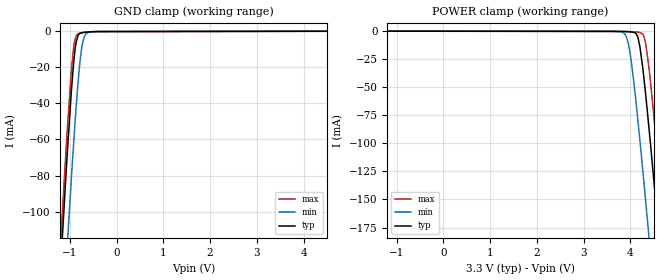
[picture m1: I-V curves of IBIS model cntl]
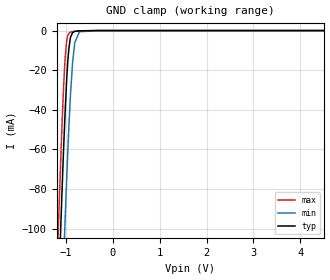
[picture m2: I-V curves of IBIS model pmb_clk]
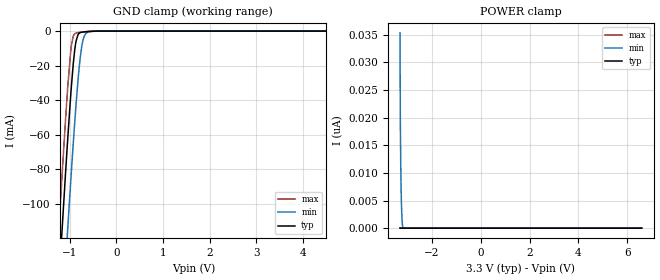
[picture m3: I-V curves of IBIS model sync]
|Texas Instruments Incorporated
| TPS40400 3.0-V TO 20-V PMBus SYNCHRONOUS BUCK CONTROLLER
| Marketing part#   Digital Voltage Range   Package-type   #pins
| TPS40400RHLR   3.0V-3.4V   VQFN   24
| TPS40400RHLT   3.0V-3.4V   VQFN   24
[IBIS Ver]   4.1
[File name]   tps40400.ibs
[File Rev]   2.0
[Date]   4/17/2015
[Source]
| Texas Instruments Incorporated.
| Analog-eLab Design Center, HPA
| 12500 TI Blvd
| Dallas, TX -75243
[Notes]   Revision History:
| Rev 2.0: 4/17/2015
| - New models added for CNTL, PGOOD and SYNC.
| Rev 1.1: 7/1/2013
| - Modeled with respect to different V_fixture voltages
| Rev 1.0: 6/21/2013
| - Initial version of the model
| - Model generated from simulations in TISPICE
| - Model matched to SPICE simulation
| - C_comp although listed in numerical order of value are
|   obtained from varying PVT conditions. For PVT conditions for
|   each specific value refer the buffer description under
|   respective [Model]. IBIS model user is responsible for using
|   appropriate C_comp to simulate for Signal Integrity.
|*  EXCEPTION:   *
|*  - For model sync, there will be a leakage current in the Ground Clamp   *
|*   I-V Table because of the pulldown transistors MN0 and MN1 in ESD   *
|*   connected to pad.   *
|*  - For model pgood, there will be a leakage current in the Power Clamp   *
|*   I-V Table because of the MP1 and MN1 transistors in the BU140 block   *
|*   connected to pad.End points do not match fixture voltages due to the   *
|*   pull up resistance (100kohms)  connected to the pad.   *
|*  - For model smbalrt, there will be a leakage current in the Power Clamp  *
|*   I-V Table because of the transistor MN1 in PGOOD_FET block connected   *
|*   to pad.   *
|*  - For model data, there will be a leakage current in the Power Clamp   *
|*   I-V Table because of the transistor (MN0, MN1) and diode (XDD0) in   *
|*   ESD block  connected to pad.   *
[Disclaimer]
| This model is designed as an aid for customers of Texas Instruments.
| TI and its licensors and suppliers make no warranties, either expressed
| or implied, with respect to this  model, including the warranties of
| merchantability or fitness for a particular purpose. The model is
| provided solely on an "as is" basis. The entire risk as to its quality
| and performance is with the customer.
[Copyright]
(C) Copyright 2015 Texas Instruments Incorporated.All rights reserved.
|   TPS540400
[Component]   TPS540400
[Manufacturer]   TI
[Package]   |24 VQFN
|   typ   min   max
R_pkg  0.042266   0.000540  0.065360
L_pkg  0.707532nH 0.114770nH 1.090470nH
C_pkg  0.120390pF 0.069160pF 0.145430pF
[Pin]  signal_name   model_name   R_pin   L_pin   C_pin
1   CLK   pmb_clk   NA   NA   NA
2   CNTL   cntl   NA   NA   NA
3   PGOOD   pgood   NA   NA   NA
4   SYNC   sync   NA   NA   NA
5   TRACK   NC   NA   NA   NA
6   COMP   NC   NA   NA   NA
7   FB   NC   NA   NA   NA
8   DIFFO   NC   NA   NA   NA
9   VSNS+   NC   NA   NA   NA
10   VSNS-   NC   NA   NA   NA
11   ISNS-   NC   NA   NA   NA
12   ISNS+   NC   NA   NA   NA
13   BP3   NC   NA   NA   NA
14   BP6   NC   NA   NA   NA
15   GND   GND   NA   NA   NA
16   LDRV   NC   NA   NA   NA
17   SW   NC   NA   NA   NA
18   BOOT   NC   NA   NA   NA
19   HDRV   NC   NA   NA   NA
20   VDD   POWER   NA   NA   NA
21   ADDR0   nc   NA   NA   NA
22   ADDR1   nc   NA   NA   NA
23   SMBALRT   smbalrt   NA   NA   NA
24   DATA   data   NA   NA   NA
|   Model Selectors
[Model Selector] data
data_pr_5   3.3V digital I/O_open_drain with V_fixture = 5V
data_pr_3p3 3.3V digital I/O_open_drain with V_fixture = 3.3V
data_pr_1p8 3.3V digital I/O_open_drain with V_fixture = 1.8V
[Model Selector] smbalrt
smbalrt_pr_5   3.3V digital open_sink with V_fixture = 5V
smbalrt_pr_3p3 3.3V digital open_sink with V_fixture = 3.3V
smbalrt_pr_1p8 3.3V digital open_sink with V_fixture = 1.8V
[Model Selector] pgood
pgood_pr_5   3.3V digital open_sink with V_fixture = 5V
pgood_pr_3p3 3.3V digital open_sink with V_fixture = 3.3V
pgood_pr_1p8 3.3V digital open_sink with V_fixture = 1.8V
| Models and submodels in the file (12): cntl (Input), pmb_clk (Input), sync (Input), smbalrt_pr_1p8 (Open_sink), smbalrt_pr_3p3 (Open_sink), smbalrt_pr_5 (Open_sink), data_pr_1p8 (I/O_open_drain), data_pr_3p3 (I/O_open_drain), data_pr_5 (I/O_open_drain), pgood_pr_5 (Open_drain), pgood_pr_3p3 (Open_drain), pgood_pr_1p8 (Open_drain)
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|   cntl Model
[Model]   cntl
Model_type   Input
Vinl = 0.8
Vinh = 2.1
|   typ   min   max
C_comp   0.176pF   0.150pF   0.210pF
[Voltage Range]   3.3   3.2   3.4
[Temperature Range]   25   125   -40
[Power Clamp Reference]   3.3   3.2   3.4
[GND Clamp Reference]   -0   -0   -0
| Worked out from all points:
|   GND clamp passes 1 mA (typ) near -0.73 V on its own axis
[GND Clamp]
|   Voltage   I(typ)   I(min)   I(max)
-3.3V     -1.154A    -1.202A    -1.142A
-1.231V   -146.1mA   -198.6mA   -132.5mA
-1.092V   -84.06mA   -135.8mA   -70.75mA
-1.043V   -63.1mA    -114.1mA   -50.17mA
-973.5mV  -35.96mA   -84.64mA   -24.42mA
-924mV    -19.54mA   -64.6mA    -10.6mA
-864.6mV  -6.393mA   -42.31mA   -2.848mA
-815.1mV  -2.251mA   -26.11mA   -1.478mA
-755.7mV  -1.16mA    -11.44mA   -1.108mA
-706.2mV  -923.4uA   -4.598mA   -948.2uA
-547.8mV  -553.6uA   -646.5uA   -584.9uA
6.59V     -180.4uA   -165uA     -204.1uA
[POWER Clamp]
|   Voltage   I(typ)   I(min)   I(max)
-3.3V     -180uA     -168.1uA   -199.9uA
3.818V    -509.1uA   -1.084mA   -476.1uA
3.917V    -688.3uA   -5.682mA   -541.7uA
3.986V    -861.9uA   -18.23mA   -654.3uA
4.125V    -2.705mA   -64.99mA   -1.004mA
4.204V    -14.18mA   -97.53mA   -1.371mA
4.293V    -43.35mA   -136.3mA   -5.351mA
4.333V    -59.03mA   -154mA     -12.65mA
4.402V    -88.35mA   -185.4mA   -34.47mA
4.6V      -178.2mA   -277.5mA   -118.5mA
4.788V    -266.9mA   -366.7mA   -206mA
6.59V     -1.149A    -1.247A    -1.087A
|   pmb_clk Model
[Model]   pmb_clk
Model_type   Input
Vinl = 0.8
Vinh = 2.1
|   typ   min   max
|   (nom PVT)   (fast PVT)   (slow PVT)
C_comp   5.652e-14   5.542e-14   5.833e-14
| Where nom  PVT is Nominal Process, 3.3V, 25C
|   Fast PVT is Strong Process,  3.4V, -40C
|   Slow PVT is Weak Process,   3.2V, 125C
[Voltage Range]   3.3   3.2   3.4
|Junction Temperature
[Temperature Range]   25   125   -40
[Power Clamp Reference]   3.3   3.2   3.4
[GND Clamp Reference]   0   0   0
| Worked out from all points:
|   GND clamp passes 1 mA (typ) near -0.85 V on its own axis
[GND Clamp]
|   Voltage   I(typ)   I(min)   I(max)
-3.3V     -1.871A    -1.918A    -1.848A
-1.175V   -145.3mA   -205mA     -109.9mA
-1.158V   -133.2mA   -192.9mA   -97.97mA
-1.143V   -122.5mA   -182mA     -87.34mA
-1.09V    -85.9mA    -144.4mA   -51.94mA
-1.025V   -45.95mA   -101.1mA   -17.51mA
-960.8mV  -16mA      -61.8mA    -2.658mA
-904.2mV  -3.714mA   -33.19mA   -823.8uA
-858.4mV  -1.052mA   -16.34mA   -532uA
-813.6mV  -421.3uA   -6.609mA   -368.5uA
-711.2mV  -114.9uA   -593.5uA   -127.1uA
6.6V      0A         0A         0A
[POWER Clamp]
|   Voltage   I(typ)   I(min)   I(max)
-3.3V     0A         0A         0A
0V        0A         0A         0A
6.6V      0A         0A         0A
|   sync Model
[Model]   sync
Model_type   Input
Vinl = 0.8
Vinh = 2.1
|   typ   min   max
C_comp   0.254pF   0.192pF   0.296pF
[Voltage Range]   3.3   3.2   3.4
[Temperature Range]   25   125   -40
[Power Clamp Reference]   3.3   3.2   3.4
[GND Clamp Reference]   -0   -0   -0
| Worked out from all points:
|   GND clamp passes 1 mA (typ) near -0.78 V on its own axis
[GND Clamp]
|   Voltage   I(typ)   I(min)   I(max)
-3.3V     -1.153A    -1.202A    -1.125A
-1.27V    -163.3mA   -216.8mA   -131.5mA
-1.231V   -145.1mA   -198.6mA   -113.2mA
-1.181V   -122.5mA   -175.9mA   -90.69mA
-1.043V   -62.05mA   -114.1mA   -32.13mA
-963.6mV  -31.42mA   -80.49mA   -7.98mA
-864.6mV  -5.721mA   -42.2mA    -1.132mA
-795.3mV  -1.222mA   -20.35mA   -772.9uA
-735.9mV  -633.4uA   -7.834mA   -563.9uA
-676.5mV  -427.5uA   -2.263mA   -379.5uA
-577.5mV  -196.6uA   -391.3uA   -137.4uA
6.59V     0A         0A         0A
[POWER Clamp]
|   Voltage   I(typ)   I(min)   I(max)
-3.3V     44.8pA     35.31nA    23.59pA
-3.29V    22.4pA     21.23nA    11.79pA
-3.28V    0A         15.65nA    0A
-3.27V    0A         11.46nA    0A
-3.26V    0A         8.325nA    0A
-3.251V   0A         5.971nA    0A
-3.241V   0A         4.205nA    0A
-3.221V   0A         1.887nA    0A
-3.211V   0A         1.141nA    0A
-3.191V   0A         160pA      0A
-3.171V   0A         0A         0A
6.59V     0A         0A         0A
